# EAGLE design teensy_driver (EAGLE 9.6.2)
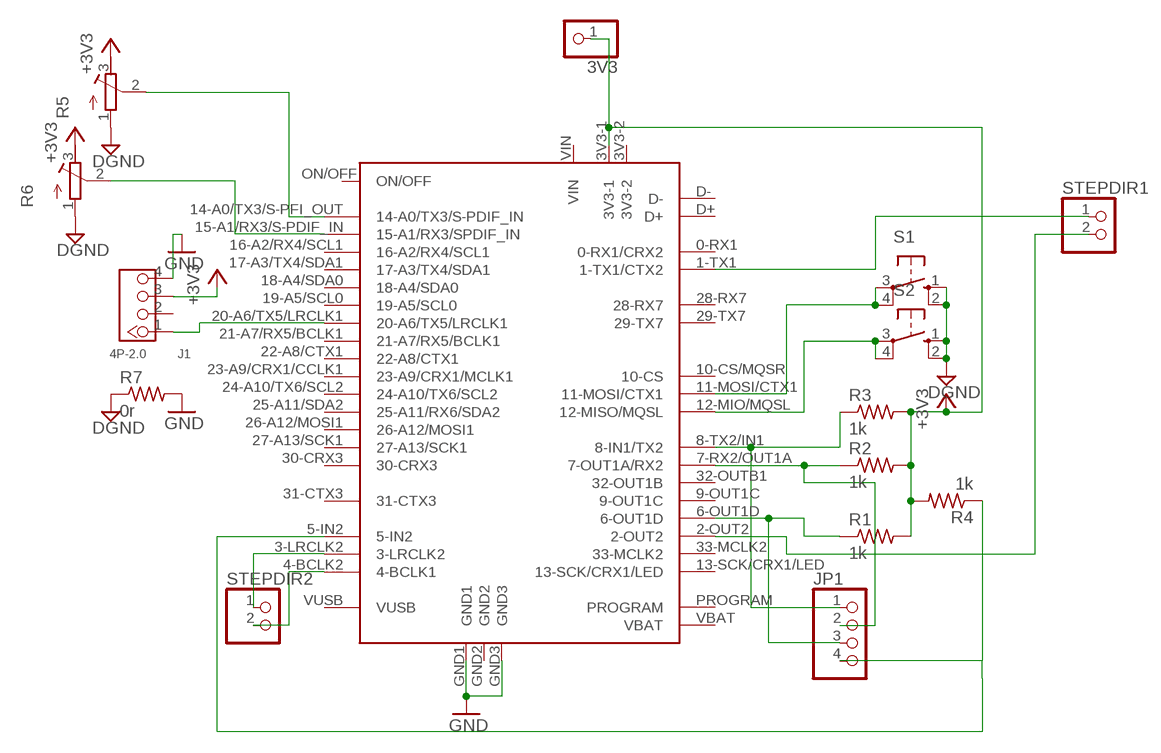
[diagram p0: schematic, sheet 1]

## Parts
3V3  PINHD-1X1  [1X01]
J1  4P-2.0  GROVE-CONNECTOR-DIP(4P-2.0)  [HW4-2.0]
JP1  PINHD-1X4  [1X04]
R1  1k  R-US_0207/7  [0207/7]
R2  1k  R-US_0207/7  [0207/7]
R3  1k  R-US_0207/7  [0207/7]
R4  1k  R-US_0207/7  [0207/7]
R5  R-TRIMM74X  [RTRIM74X]
R6  R-TRIMM74X  [RTRIM74X]
R7  0r  R-US_0204/7  [0204/7]
S1  10-XX  [B3F-10XX]
S2  10-XX  [B3F-10XX]
STEPDIR1  PINHD-1X2  [1X02]
STEPDIR2  PINHD-1X2  [1X02]
U$1  TEENSY40  [TEENSY40]

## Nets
+3V3: 3V3.1 J1.3 R1.2 R2.2 R3.2 R4.2 R5.3(E) R6.3(E) U$1.3V3-1
DGND: R5.1(A) R6.1(A) R7.1 S1.1(S) S1.2(S1) S2.1(S) S2.2(S1)
GND: J1.4 R7.2 U$1.GND1 U$1.GND3
N$1: JP1.3 R1.1 U$1.6-OUT1D
N$2: JP1.2 R2.1 U$1.7-RX2/OUT1A(7-OUT1A/RX2)
N$3: JP1.1 R3.1 U$1.8-TX2/IN1(8-IN1/TX2)
N$4: JP1.4 R4.1 U$1.5-IN2
N$5: STEPDIR1.2 U$1.2-OUT2
N$6: STEPDIR1.1 U$1.1-TX1(1-TX1/CTX2)
N$7: STEPDIR2.1 U$1.3-LRCLK2
N$8: STEPDIR2.2 U$1.4-BCLK2(4-BCLK1)
N$9: J1.1 U$1.20-A6/TX5/LRCLK1
N$10: R5.2(S) U$1.14-A0/TX3/S-PFI_OUT(14-A0/TX3/S-PDIF_IN)
N$11: R6.2(S) U$1.15-A1/RX3/S-PDIF_IN(15-A1/RX3/SPDIF_IN)
N$12: S1.3(P) S1.4(P1) U$1.11-MOSI/CTX1
N$13: S2.3(P) S2.4(P1) U$1.12-MIO/MQSL(12-MISO/MQSL)
Unconnected: J1.2 U$1.0-RX1(0-RX1/CRX2) U$1.3V3-2 U$1.9-OUT1C U$1.10-CS/MQSR(10-CS) U$1.13-SCK/CRX1/LED U$1.16-A2/RX4/SCL1 U$1.17-A3/TX4/SDA1 U$1.18-A4/SDA0 U$1.19-A5/SCL0 U$1.21-A7/RX5/BCLK1 U$1.22-A8/CTX1 U$1.23-A9/CRX1/CCLK1(23-A9/CRX1/MCLK1) U$1.24-A10/TX6/SCL2 U$1.25-A11/SDA2(25-A11/RX6/SDA2) U$1.26-A12/MOSI1 U$1.27-A13/SCK1 U$1.28-RX7 U$1.29-TX7 U$1.30-CRX3 U$1.31-CTX3 U$1.32-OUTB1(32-OUT1B) U$1.33-MCLK2 U$1.D+ U$1.D- U$1.GND2 U$1.ON/OFF U$1.PROGRAM U$1.VBAT U$1.VIN U$1.VUSB

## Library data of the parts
3V3 = pinhead:PINHD-1X1: PIN HEADER
J1 = OPL_Connector:GROVE-CONNECTOR-DIP(4P-2.0): 320110033
JP1 = pinhead:PINHD-1X4: PIN HEADER
R1-R4 R7 = rcl:R-US_: RESISTOR, American symbol; SPICEPREFIX: R
R5 R6 = rcl:R-TRIMM: Trimm resistor; SPICEMODEL: X; SPICEPREFIXL: POT
S1 S2 = switch-omron:10-XX: OMRON SWITCH; MPN: B3F-1000; OC_FARNELL: 176432; OC_NEWARK: 36M3542
STEPDIR1 STEPDIR2 = pinhead:PINHD-1X2: PIN HEADER
U$1 = teensy:TEENSY40: Teensy 4.0 device including POGO pins for pins 24 - 33, but not yet pins for D+ and D-. Symbol layout is what works for me and may not suite everyone... that can be added or additional symbols can be created to be used in a modilied davie name.

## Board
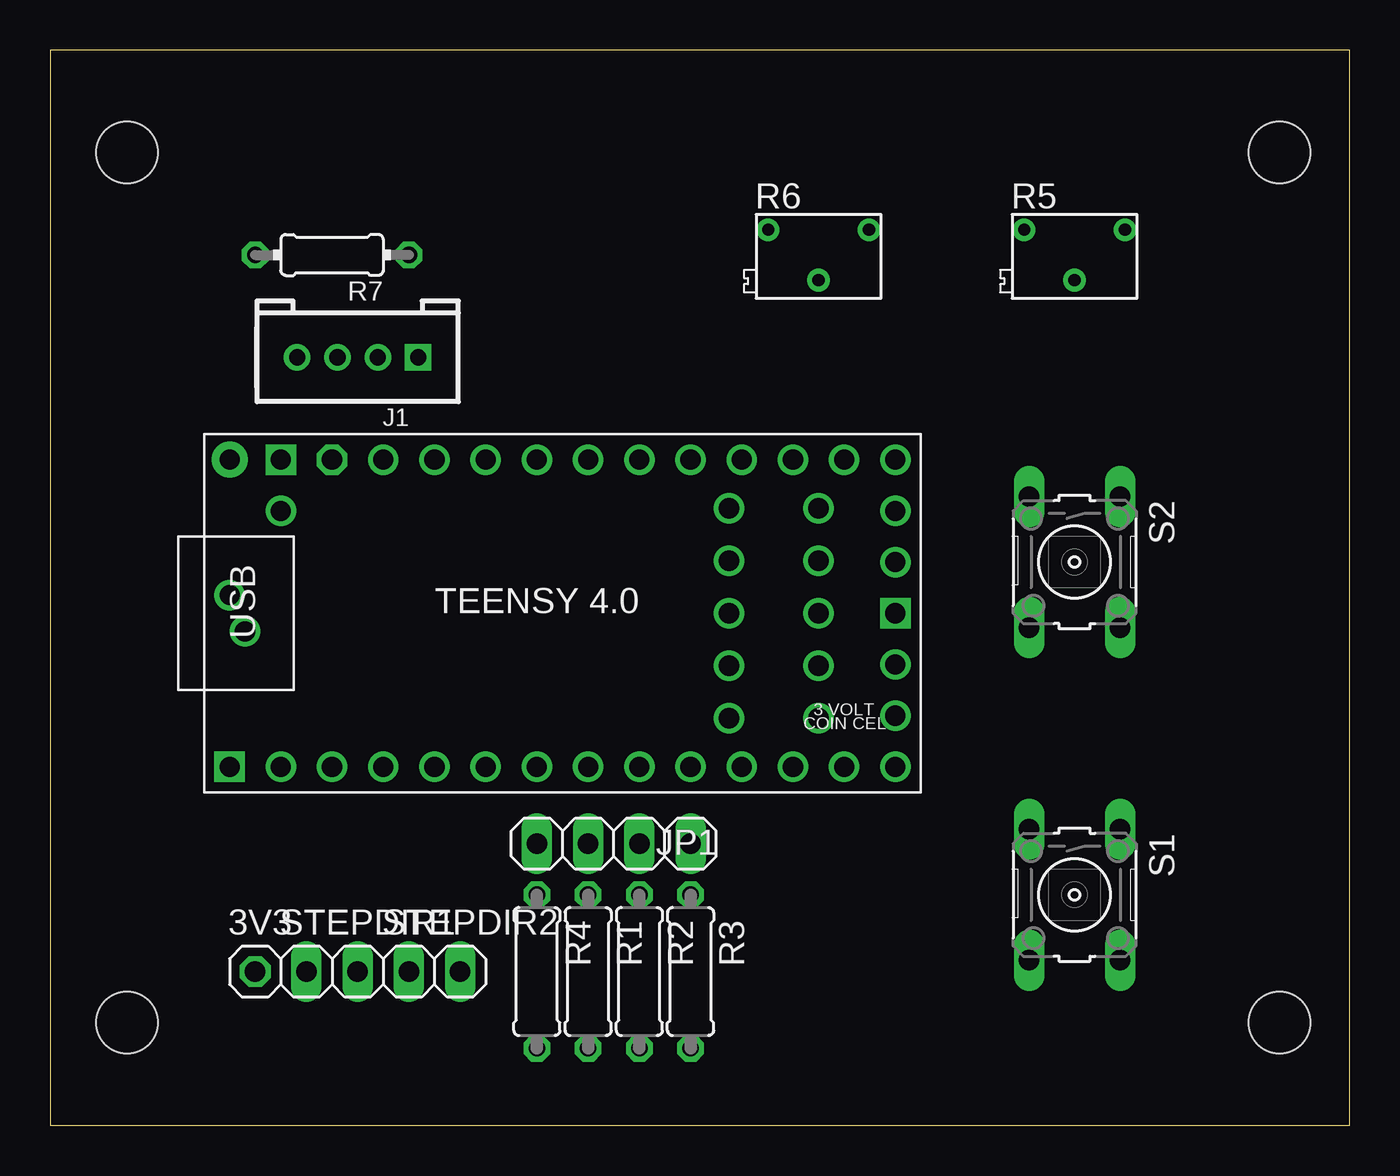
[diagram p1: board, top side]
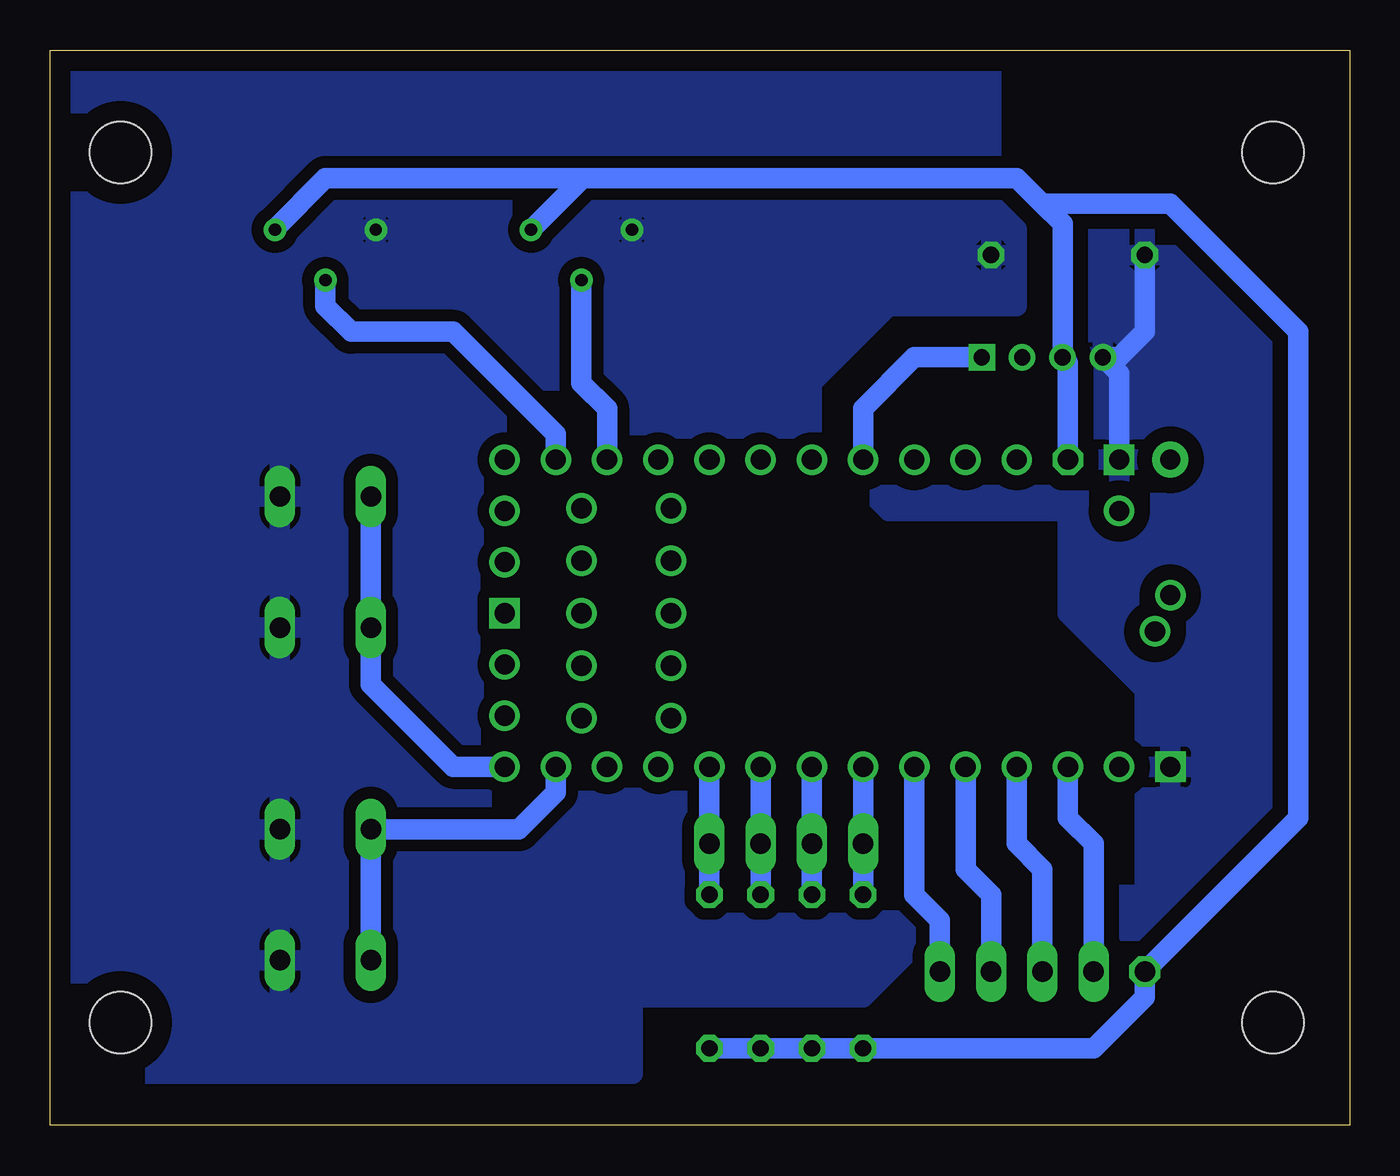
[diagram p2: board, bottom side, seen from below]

Size 64.44 x 53.33 mm. Coordinates in mm from the lower left corner, seen from the top.
Outline: 0,0 64.44,0 64.44,53.33 0,53.33 0,0
Copper layers (1*16): Top 0.035mm / dielectric 1.5mm / Bottom 0.035mm
Design rules "default": minimum track width 6mil, minimum drill 0.35mm, track to track 6mil, track to pad 6mil, pad to pad 6mil, via to via 6mil, smd to smd 6mil, copper to edge 40mil, drill to drill 6mil, minimum pad ring 10mil, minimum via ring 8mil, stop-mask expansion 4mil, vias tented up to drill 0mil, thermal gap 10mil
Holes 3.05 mm at 3.81,48.26 60.96,48.26 60.96,5.08 3.81,5.08

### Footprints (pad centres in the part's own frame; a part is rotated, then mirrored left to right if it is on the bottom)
1X01 = drill 1.016 octagon: 1 0,0
HW4-2.0 = drill 0.8 pad 1.27 square: 1 -3,0 | drill 0.8 pad 1.27: 2 -1,0; 3 1,0; 4 3,0
1X04 = drill 1.016 long: 1 -3.81,0; 2 -1.27,0; 3 1.27,0; 4 3.81,0
0207/7 = drill 0.813 octagon: 1 -3.81,0; 2 3.81,0
RTRIM74X = drill 0.61: 1 -1.25,-2.5; 2 1.25,0; 3 -1.25,2.5
0204/7 = drill 0.813 octagon: 1 -3.81,0; 2 3.81,0
B3F-10XX = drill 1.016 long: 1 -3.251,2.261; 2 3.251,2.261; 3 -3.251,-2.261; 4 3.251,-2.261
1X02 = drill 1.016 long: 1 -1.27,0; 2 1.27,0
TEENSY40 = drill 1: 0-RX1 -13.97,-7.62; 1-TX1 -11.43,-7.62; 2-OUT2 -8.89,-7.62; 3-LRCLK2 -6.35,-7.62; 3V3-2 16.51,-2.54; 4-BCLK2 -3.81,-7.62; 5-IN2 -1.27,-7.62; 6-OUT1D 1.27,-7.62; 7-RX2/OUT1A 3.81,-7.62; 8-TX2/IN1 6.35,-7.62; 9-OUT1C 8.89,-7.62; 10-CS/MQSR 11.43,-7.62; 11-MOSI/CTX1 13.97,-7.62; 12-MIO/MQSL 16.51,-7.62; 13-SCK/CRX1/LED 16.51,7.62; 14-A0/TX3/S-PFI_OUT 13.97,7.62; 15-A1/RX3/S-PDIF_IN 11.43,7.62; 16-A2/RX4/SCL1 8.89,7.62; 17-A3/TX4/SDA1 6.35,7.62; 18-A4/SDA0 3.81,7.62; 19-A5/SCL0 1.27,7.62; 20-A6/TX5/LRCLK1 -1.27,7.62; 21-A7/RX5/BCLK1 -3.81,7.62; 22-A8/CTX1 -6.35,7.62; 23-A9/CRX1/CCLK1 -8.89,7.62; 24-A10/TX6/SCL2 12.7,5.207; 25-A11/SDA2 8.255,5.207; 26-A12/MOSI1 12.7,2.603; 27-A13/SCK1 8.255,2.603; 28-RX7 12.7,0; 29-TX7 8.255,0; 30-CRX3 12.7,-2.603; 31-CTX3 8.255,-2.603; 32-OUTB1 12.7,-5.207; 33-MCLK2 8.255,-5.207; D+ -15.75,-0.9; D- -16.51,0.9; ON/OFF 16.51,5.08; PROGRAM 16.51,2.54; VBAT 16.51,-5.08; VUSB -13.97,5.08 | drill 1 octagon: 3V3-1 -11.43,7.62 | drill 1 square: GND1 -16.51,-7.62; GND2 16.51,0; GND3 -13.97,7.62 | drill 1 pad 1.778: VIN -16.51,7.62

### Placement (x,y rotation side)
3V3  10.16,7.62 0 top
J1  15.24,38.1 180 top
JP1  27.94,13.97 180 top
R1  26.67,7.62 270 top
R2  29.21,7.62 270 top
R3  31.75,7.62 270 top
R4  24.13,7.62 270 top
R5  50.8,43.18 270 top
R6  38.1,43.18 270 top
R7  13.97,43.18 180 top
S1  50.8,11.43 270 top
S2  50.8,27.94 270 top
STEPDIR1  13.97,7.62 0 top
STEPDIR2  19.05,7.62 0 top
U$1  25.4,25.4 0 top

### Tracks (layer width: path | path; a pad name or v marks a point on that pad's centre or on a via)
+3V3
  Bottom 1.016: U$1.3V3-1 13.97,37.83 J1.3 14.24,44.72 15.24,45.72 | R3.2 R2.2 R1.2 R4.2 12.7,3.81 10.16,6.35 3V3.1 2.54,15.24 2.54,39.37 8.89,45.72 15.24,45.72 | R6.3 38.04,46.99 | 15.24,45.72 16.51,46.99 38.04,46.99 | 38.04,46.99 50.8,46.99 53.3,44.49 R5.3
DGND
  pour Bottom (isolate 0.584): 17.78,50.8 17.78,45.72 16.51,44.45 16.51,40.64 22.86,40.64 26.67,36.83 26.67,31.75 24.13,29.21 15.24,29.21 15.24,24.13 11.43,20.32 11.43,12.7 17.78,12.7 24.13,6.35 35.56,6.35 35.56,2.54 64.77,2.54 64.77,53.34 17.78,53.34
GND
  Bottom 1.016: U$1.GND3 11.43,37.29 J1.4 11.43,38.1 10.16,39.37 R7.2
  pour Bottom (isolate 0.762, rank 2): 0,53.34 16.51,53.34 16.51,46.99 16.51,45.72 15.24,44.45 15.24,39.37 21.59,39.37 25.4,35.56 25.4,33.02 22.86,30.48 13.97,30.48 13.97,26.67 13.97,25.4 10.16,21.59 10.16,11.43 16.51,11.43 22.86,5.08 34.29,5.08 34.29,1.27 1.27,1.27 1.27,52.07
N$1
  Bottom 1.016: U$1.6-OUT1D JP1.3 R1.1
N$2
  Bottom 1.016: U$1.7-RX2/OUT1A JP1.2 R2.1
N$3
  Bottom 1.016: U$1.8-TX2/IN1 JP1.1 R3.1
N$4
  Bottom 1.016: U$1.5-IN2 JP1.4 R4.1
N$5
  Bottom 1.016: U$1.2-OUT2 16.51,13.97 15.24,12.7 STEPDIR1.2
N$6
  Bottom 1.016: STEPDIR1.1 12.7,13.97 13.97,15.24 U$1.1-TX1
N$7
  Bottom 1.016: U$1.3-LRCLK2 19.05,12.7 17.78,11.43 STEPDIR2.1
N$8
  Bottom 1.016: STEPDIR2.2 20.32,10.16 21.59,11.43 U$1.4-BCLK2
N$9
  Bottom 1.016: J1.1 21.59,38.1 24.13,35.56 U$1.20-A6/TX5/LRCLK1
N$10
  Bottom 1.016: U$1.14-A0/TX3/S-PFI_OUT 39.37,34.29 44.45,39.37 49.53,39.37 50.8,40.64 R5.2
N$11
  Bottom 1.016: R6.2 38.1,36.83 36.83,35.56 U$1.15-A1/RX3/S-PDIF_IN
N$12
  Bottom 1.016: U$1.11-MOSI/CTX1 39.37,16.51 41.2,14.68 S1.3 S1.4
N$13
  Bottom 1.016: U$1.12-MIO/MQSL 44.45,17.78 48.54,21.87 S2.4 S2.3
